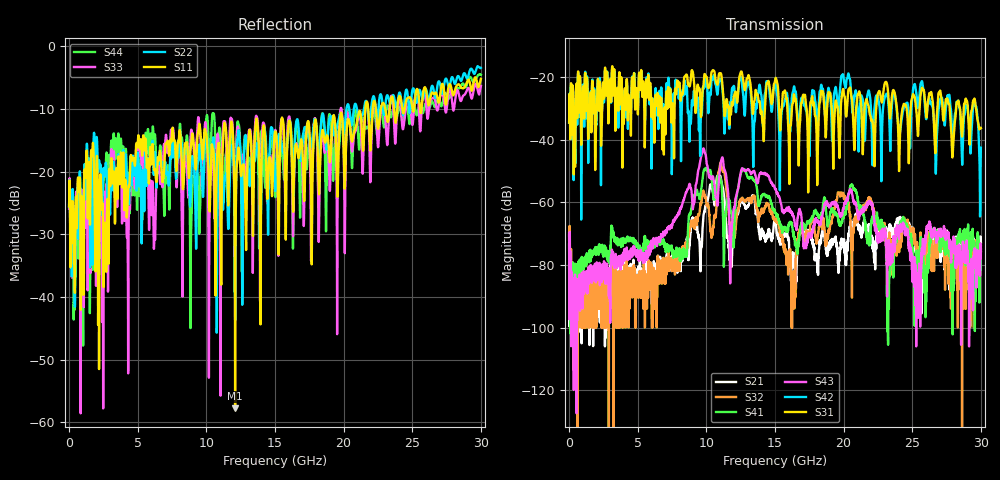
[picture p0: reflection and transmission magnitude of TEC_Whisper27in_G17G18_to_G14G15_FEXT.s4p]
! Tyco Electronics
! G17G18-G14G15_FEXT
!! PART DESCRIPTION: Whisper 27in Megtron 6 VLP-HVLP-VLP Channel Model, bulkhead 2.4mm test pts
!! MODEL DESCRIPTION: System 4-port S-parameter
!! MODEL STATUS: Measured
!! MODEL GEOMETRY: Channel Model
!! MODEL FREQUENCY RANGE: DC to 30.000 GHz in 10.000 MHz frequency steps
!! MODEL EDGE RATE LIMITATION: 12.500 ps (Using conservative 0.5/Fmax rule of thumb)
!! TIME-DOMAIN TRANSFORM CAUTIONS:
!! 1.) Do not simulate transient edge rates faster than the number listed above.  Edge rates faster than this number
!!  contain significant spectral content at frequencies above the model's highest frequency.
!! 2.) Even when simulating edge rates that are slower than the number listed above, be aware that the best time
!!  resolution possible with a direct iFFT is (1 / 2Fmax).  As a result, time resolution is typically not adequate
!!  for most time-domain simulations unless tricks such as windowing are used to minimize leakage and aliasing.
!! 3.) Because the model has a uniform frequency step, a direct iFFT will result in an impulse that that has a time
!!  length given by either (1 / Fstep) or (1 / 2Fstep), depending on the transform being used.  Care has been taken
!!  in selecting the frequency step to ensure a settled impulse response for the model.  Therefore, convolution with
!!  the model's impulse response should present no issues.  However, if directly concatenating s-parameter models
!!  in the frequency domain a user must either interpolate necessary interim frequencies or complete impulse response
!!  zero-padding.  Impulse response zero-padding is more difficult, but more accurate.
!! PORT DEFINITIONS:
!! Port  1  ----->  Side A  G17  G14  Side B  <-----  Port  2
!! Port  3  ----->  Side A  G18  G15  Side B  <-----  Port  4
! Point-to-Point link (differential)  !
! Connectors:  !
!  1: STRADA Whisper  !
! Materials:  !
!  Backplane: Megtron-6 HVLP  !
!  Daughtercard: Megtron-6 VLP  !
! Stack-up:  !
!  Backplane: 20 layers, 200mil thick  !
!  Daughtercard: 14 layers, 110mil thick  !
! Trace Length:  !
!  Backplane: 17in  !
!  Daightercards: 5in  !
! Trace Width:  !
!  Backplane: 8-13-8 mils  !
!  Daughtercards: 6-9-6 mils  !
! Geometry:  !
!  Backplane: Stripline  !
!  Daughtercards: Stripline  !
! Freq. Range: 0 GHz - 30 GHz  !
! Note1: non-mixed-mode s-parameters  !
! Note2: channel includes 2.4mm test points  !
! Touchstone data converted from IdEM dataset
# GHz S MA R 50
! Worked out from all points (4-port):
!   3000 points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, 10 MHz to 30 GHz, reference 50 ohm
!   strongest paths, dB at 10 MHz, 7.51 GHz, 15.01 GHz, 22.51 GHz, 30 GHz:
!     S31: -34.5, -28.3, -21.1, -25.2, -36.3
!     S42: -34.5, -40.8, -22.7, -26.3, -42.6
!     S43: -69.9, -67.4, -55.8, -71.7, -75.0
!     S41: -80.2, -75.4, -63.4, -65.3, -74.0
!     S32: -70.5, -81.9, -66.0, -66.4, -75.9
!     S21: -73.5, -77.9, -66.3, -68.8, -73.2
!   lowest |S11| = -57.8 dB at 12.1 GHz (marker M1), VSWR 1.00, Z = 50.1 - j0.101 ohm
!   |S11| at or under -10 dB: start of sweep to 21.59 GHz; 21.79 GHz to 22.12 GHz (324.7 MHz wide, 1.48 % of centre); 22.35 GHz to 22.71 GHz (360.6 MHz wide, 1.6 % of centre)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
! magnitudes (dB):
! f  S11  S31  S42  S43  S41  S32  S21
! 10 MHz  -25.5  -34.5  -34.5  -69.9  -80.2  -70.5  -73.5
! 7.96 GHz  -15.4  -23.1  -24.1  -63.4  -75.2  -79.2  -79.2
! 11.05 GHz  -26.7  -18.8  -20.6  -47.4  -52.6  -47.4  -52.0
! 12.1 GHz  -57.8  -24.9  -27.7  -59.9  -63.6  -69.9  -65.5
! 20.62 GHz  -15.2  -27.4  -30.0  -57.3  -54.6  -75.4  -67.1
! 25.7 GHz  -9.4  -23.5  -21.3  -74.7  -74.6  -75.4  -89.1
! 30 GHz  -5.2  -36.3  -42.6  -75.0  -74.0  -75.9  -73.2
